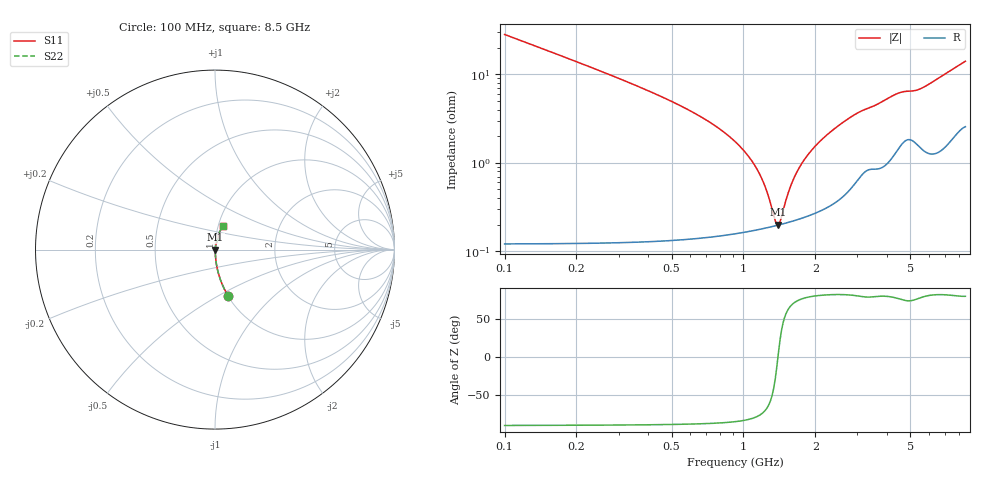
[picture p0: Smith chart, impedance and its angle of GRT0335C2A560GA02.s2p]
!Murata Part Number: GRT0335C2A560GA02
!These Parameters are Measured in Series Mode Connection
!Data Generated on Jun 19, 2026
!  o--ll--o
!Port1  Port2
!  o------o
!Operation Temp=25[degC], DC Bias Voltage=0[V]
!Freq. Start=100[MHz] Stop=9[GHz] 401[Steps]
# Hz S RI R 50
!Freq.(Hz) S11(Real) S11(Imag) S21(Real) S21(Imag) S12(Real) S12(Imag) S22(Real) S22(Imag)
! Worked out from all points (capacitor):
!   401 points, 100 MHz to 8.5 GHz, reference 50 ohm
!   read as one part in series: C = 56 pF near 142 MHz
!   lowest |Z| = 199 mohm at 1.402 GHz (marker M1)
!   series resonance near 1.395 GHz, so ESL is about 230 pH
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1e8  0.075 -0.2612  0.925 0.2612  0.925 0.2612  0.075 -0.2612
2.26e8  0.0159 -0.1203  0.9841 0.1203  0.9841 0.1203  0.0159 -0.1203
3.52e8  0.00693 -0.075  0.9931 0.075  0.9931 0.075  0.00693 -0.075
4.99e8  0.00377 -0.0494  0.9962 0.0494  0.9962 0.0494  0.00377 -0.0494
8.98e8  0.0019 -0.0185  0.9981 0.0185  0.9981 0.0185  0.0019 -0.0185
1.087e9  0.00181 -0.0102  0.9982 0.0102  0.9982 0.0102  0.00181 -0.0102
1.213e9  0.00184 -0.00571  0.9982 0.00571  0.9982 0.00571  0.00184 -0.00571
1.36e9  0.00194 -0.00103  0.9981 0.00103  0.9981 0.00103  0.00194 -0.00103
1.402e9  0.00198 0.000206  0.998 -0.000206  0.998 -0.000206  0.00198 0.000206
1.444e9  0.00202 0.00141  0.998 -0.00141  0.998 -0.00141  0.00202 0.00141
1.507e9  0.00209 0.00316  0.9979 -0.00316  0.9979 -0.00316  0.00209 0.00316
1.591e9  0.0022 0.00539  0.9978 -0.00539  0.9978 -0.00539  0.0022 0.00539
1.675e9  0.00232 0.00753  0.9977 -0.00753  0.9977 -0.00753  0.00232 0.00753
1.801e9  0.00253 0.0106  0.9975 -0.0106  0.9975 -0.0106  0.00253 0.0106
1.948e9  0.00281 0.014  0.9972 -0.014  0.9972 -0.014  0.00281 0.014
2.137e9  0.00325 0.0182  0.9968 -0.0182  0.9968 -0.0182  0.00325 0.0182
2.347e9  0.00386 0.0227  0.9961 -0.0227  0.9961 -0.0227  0.00386 0.0227
2.914e9  0.00684 0.034  0.9932 -0.034  0.9932 -0.034  0.00684 0.034
4.3e9  0.0155 0.056  0.9845 -0.056  0.9845 -0.056  0.0155 0.056
5.707e9  0.0182 0.0686  0.9818 -0.0686  0.9818 -0.0686  0.0182 0.0686
7.114e9  0.0256 0.0989  0.9744 -0.0989  0.9744 -0.0989  0.0256 0.0989
8.5e9  0.0425 0.1294  0.9575 -0.1294  0.9575 -0.1294  0.0425 0.1294
